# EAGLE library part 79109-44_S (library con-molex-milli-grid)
RECEPTACAL
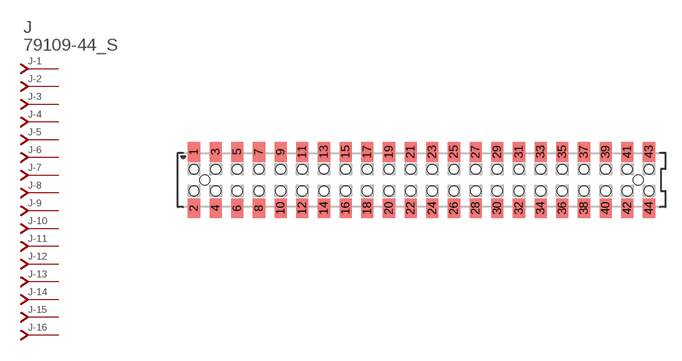
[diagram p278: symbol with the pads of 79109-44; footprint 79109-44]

Designator prefix J; gates -1=J-NV -2=J-N -3=J-N -4=J-N -5=J-N -6=J-N -7=J-N -8=J-N -9=J-N -10=J-N -11=J-N -12=J-N -13=J-N -14=J-N -15=J-N -16=J-N -17=J-N -18=J-N -19=J-N -20=J-N -21=J-N -22=J-N -23=J-N -24=J-N -25=J-N -26=J-N -27=J-N -28=J-N -29=J-N -30=J-N -31=J-N -32=J-N -33=J-N -34=J-N -35=J-N -36=J-N -37=J-N -38=J-N -39=J-N -40=J-N -41=J-N -42=J-N -43=J-N -44=J-N

## 79109-44_S  [79109-44]
1  -1:J  pas
2  -2:J  pas
3  -3:J  pas
4  -4:J  pas
5  -5:J  pas
6  -6:J  pas
7  -7:J  pas
8  -8:J  pas
9  -9:J  pas
10  -10:J  pas
11  -11:J  pas
12  -12:J  pas
13  -13:J  pas
14  -14:J  pas
15  -15:J  pas
16  -16:J  pas
17  -17:J  pas
18  -18:J  pas
19  -19:J  pas
20  -20:J  pas
21  -21:J  pas
22  -22:J  pas
23  -23:J  pas
24  -24:J  pas
25  -25:J  pas
26  -26:J  pas
27  -27:J  pas
28  -28:J  pas
29  -29:J  pas
30  -30:J  pas
31  -31:J  pas
32  -32:J  pas
33  -33:J  pas
34  -34:J  pas
35  -35:J  pas
36  -36:J  pas
37  -37:J  pas
38  -38:J  pas
39  -39:J  pas
40  -40:J  pas
41  -41:J  pas
42  -42:J  pas
43  -43:J  pas
44  -44:J  pas

## Footprint 79109-44 (pad centres in mm)
RECEPTACAL SMD Dual Row, Vertical, Pass-Thru
smd 1.12 x 1.83: 1 -21,2.6; 2 -21,-2.6; 3 -19,2.6; 4 -19,-2.6; 5 -17,2.6; 6 -17,-2.6; 7 -15,2.6; 8 -15,-2.6; 9 -13,2.6; 10 -13,-2.6; 11 -11,2.6; 12 -11,-2.6; 13 -9,2.6; 14 -9,-2.6; 15 -7,2.6; 16 -7,-2.6; 17 -5,2.6; 18 -5,-2.6; 19 -3,2.6; 20 -3,-2.6; 21 -1,2.6; 22 -1,-2.6; 23 1,2.6; 24 1,-2.6; 25 3,2.6; 26 3,-2.6; 27 5,2.6; 28 5,-2.6; 29 7,2.6; 30 7,-2.6; 31 9,2.6; 32 9,-2.6; 33 11,2.6; 34 11,-2.6; 35 13,2.6; 36 13,-2.6; 37 15,2.6; 38 15,-2.6; 39 17,2.6; 40 17,-2.6; 41 19,2.6; 42 19,-2.6; 43 21,2.6; 44 21,-2.6
hole 0.914 at -20,0
hole 0.914 at -21,1
hole 0.914 at -21,-1
hole 0.914 at -19,-1
hole 0.914 at -19,1
hole 0.914 at -17,-1
hole 0.914 at -17,1
hole 0.914 at 20,0
hole 0.914 at -15,1
hole 0.914 at -15,-1
hole 0.914 at -13,1
hole 0.914 at -13,-1
hole 0.914 at -11,1
hole 0.914 at -11,-1
hole 0.914 at -9,1
hole 0.914 at -9,-1
hole 0.914 at -7,-1
hole 0.914 at -7,1
hole 0.914 at -5,1
hole 0.914 at -5,-1
hole 0.914 at -3,1
hole 0.914 at -3,-1
hole 0.914 at -1,1
hole 0.914 at -1,-1
hole 0.914 at 1,-1
hole 0.914 at 1,1
hole 0.914 at 3,1
hole 0.914 at 5,1
hole 0.914 at 7,1
hole 0.914 at 3,-1
hole 0.914 at 5,-1
hole 0.914 at 7,-1
hole 0.914 at 9,-1
hole 0.914 at 11,-1
hole 0.914 at 13,-1
hole 0.914 at 15,-1
hole 0.914 at 17,-1
hole 0.914 at 9,1
hole 0.914 at 11,1
hole 0.914 at 13,1
hole 0.914 at 15,1
hole 0.914 at 17,1
hole 0.914 at 19,-1
hole 0.914 at 21,-1
hole 0.914 at 19,1
hole 0.914 at 21,1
